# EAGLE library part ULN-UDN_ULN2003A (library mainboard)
DRIVER ARRAY
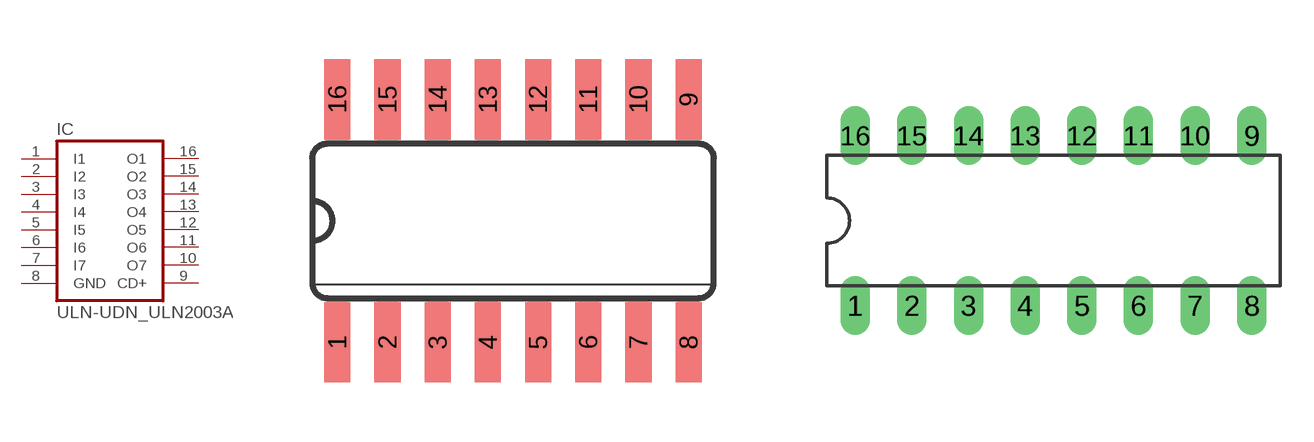
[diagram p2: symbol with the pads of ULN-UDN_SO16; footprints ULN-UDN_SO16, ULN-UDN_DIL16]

Designator prefix IC

## ULN-UDN_ULN2003AD  [ULN-UDN_SO16]
1  I1  in
2  I2  in
3  I3  in
4  I4  in
5  I5  in
6  I6  in
7  I7  in
8  GND  pwr
9  CD+  pas
10  O7  oc
11  O6  oc
12  O5  oc
13  O4  oc
14  O3  oc
15  O2  oc
16  O1  oc

## ULN-UDN_ULN2003AN  [ULN-UDN_DIL16]
Pads as for ULN-UDN_SO16

## Footprint ULN-UDN_SO16 (pad centres in mm)
Small Outline Package
smd 0.66 x 2.032: 1 -4.445,-3.073; 2 -3.175,-3.073; 3 -1.905,-3.073; 4 -0.635,-3.073; 5 0.635,-3.073; 6 1.905,-3.073; 7 3.175,-3.073; 8 4.445,-3.073; 9 4.445,3.073; 10 3.175,3.073; 11 1.905,3.073; 12 0.635,3.073; 13 -0.635,3.073; 14 -1.905,3.073; 15 -3.175,3.073; 16 -4.445,3.073

## Footprint ULN-UDN_DIL16 (pad centres in mm)
Dual In Line Package
drill 0.813 long: 1 -8.89,-3.81; 2 -6.35,-3.81; 3 -3.81,-3.81; 4 -1.27,-3.81; 5 1.27,-3.81; 6 3.81,-3.81; 7 6.35,-3.81; 8 8.89,-3.81; 9 8.89,3.81; 10 6.35,3.81; 11 3.81,3.81; 12 1.27,3.81; 13 -1.27,3.81; 14 -3.81,3.81; 15 -6.35,3.81; 16 -8.89,3.81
